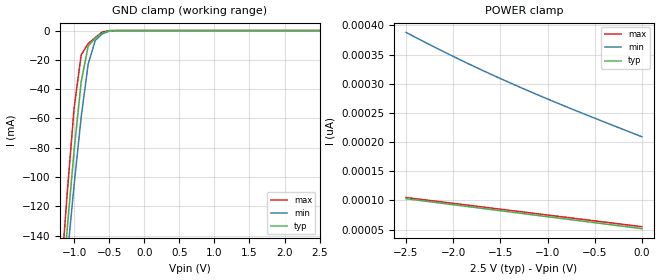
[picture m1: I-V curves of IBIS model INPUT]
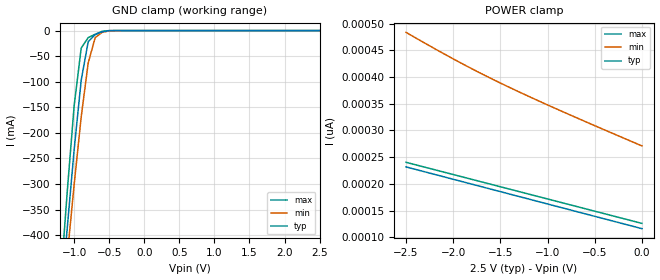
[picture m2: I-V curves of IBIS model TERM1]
|   PERICOM SEMICONDUCTOR CORP
|   IBIS Model of PI3C32X245
|   Product Family: 3C
|   BQSOP (B) Package
[IBIS Ver] 3.2
[Comment char] |_char
[File Name] pi3c32x245_b_25v.ibs
[File Rev] 2.0
[Source] File originated at Pericom Semiconductor Corp.
[Date] 03/15/18
[Disclaimer] (C) Copyright PERICOM Semiconductor Corporation
   All rights reserved
  Pericom Semiconductor Corporation hereby grants the user of
  this IBIS model a non-exclusive, nontransferable license to
  use this IBIS model under the following terms.
  This IBIS model is provided on an "AS IS" basis and Pericom
  makes absolutely no warranty with respect to the information
  contained herein. PERICOM DISCLAIMS AND CUSTOMER WAIVES ALL
  WARRANTIES, EXPRESSED OR IMPLIED, INCLUDING WARRANTIES OF
  MERCHANTABILITY OR FITNESS FOR A PARTICULAR PURPOSE. The
  entire risk as to quality and performance is with the customer.
  Accordingly, in no event shall the company be liable for any
  damages, whether in contract or tort, including any lost
  profits or other incidental, consequential, exemplary, or
  punitive damages arising out of the use or application of the
  IBIS model provided in this package. Further, Pericom reserves
  the right to make changes without notice to any product herein
  to improve reliability, function, or design. Pericom does not
  convey any license under patent rights or any other intellectual
  property rights, including those of third parties.
  The user is granted this license only to use the IBIS model
  and is not granted rights to sell, load, rent, lease or license
  the IBIS model in whole or in part, or in modified form to anyone
  other than user. User may modify the IBIS model to suit its specific
  application but rights to derivative works and such modifications
  shall belong to Pericom.
  Pericom is not obligated to provide maintenance or support
  for the licensed IBIS model.
  Contact Pericom at ATTN: APPLICATION ENGINEERING / IBIS MODELS
  2380 Bering Drive, San Jose, CA 95131
[Component] PI3C32X245
[Manufacturer] Pericom Semiconductor Corp.
[Package]
| Variable   typ   min   max
R_pkg   0.03818ohm   0.02666ohm   0.04970ohm
L_pkg   0.79246nH   0.73792nH   0.84700nH
C_pkg   0.19953pF   0.16164pF   0.23742pF
[Pin]  signal_name   model_name   R_pin   L_pin   C_pin
1   NC   NC   0.04970   0.84700nH   0.23742pF
2   A0   TERM1   0.04714   0.83488nH   0.22900pF
3   A1   TERM1   0.04458   0.82276nH   0.22058pF
4   A2   TERM1   0.04202   0.81064nH   0.21216pF
5   A3   TERM1   0.03946   0.79852nH   0.20374pF
6   A4   TERM1   0.03690   0.78640nH   0.19532pF
7   A5   TERM1   0.03434   0.77428nH   0.18690pF
8   A6   TERM1   0.03178   0.76216nH   0.17848pF
9   A7   TERM1   0.02922   0.75004nH   0.17006pF
10   GND   GND   0.02666   0.73792nH   0.16164pF
11   NC   NC   0.02666   0.73792nH   0.16164pF
12   A8   TERM1   0.02922   0.75004nH   0.17006pF
13   A9   TERM1   0.03178   0.76216nH   0.17848pF
14   A10   TERM1   0.03434   0.77428nH   0.18690pF
15   A11   TERM1   0.03690   0.78640nH   0.19532pF
16   A12   TERM1   0.03946   0.79852nH   0.20374pF
17   A13   TERM1   0.04202   0.81064nH   0.21216pF
18   A14   TERM1   0.04458   0.82276nH   0.22058pF
19   A15   TERM1   0.04714   0.83488nH   0.22900pF
20   GND   GND   0.04970   0.84700nH   0.23742pF
21   B15   TERM2   0.04970   0.84700nH   0.23742pF
22   B14   TERM2   0.04714   0.83488nH   0.22900pF
23   B13   TERM2   0.04458   0.82276nH   0.22058pF
24   B12   TERM2   0.04202   0.81064nH   0.21216pF
25   B11   TERM2   0.03946   0.79852nH   0.20374pF
26   B10   TERM2   0.03690   0.78640nH   0.19532pF
27   B9   TERM2   0.03434   0.77428nH   0.18690pF
28   B8   TERM2   0.03178   0.76216nH   0.17848pF
29   _BE2   INPUT   0.02922   0.75004nH   0.17006pF
30   VCC   POWER   0.02666   0.73792nH   0.16164pF
31   B7   TERM2   0.02666   0.73792nH   0.16164pF
32   B6   TERM2   0.02922   0.75004nH   0.17006pF
33   B5   TERM2   0.03178   0.76216nH   0.17848pF
34   B4   TERM2   0.03434   0.77428nH   0.18690pF
35   B3   TERM2   0.03690   0.78640nH   0.19532pF
36   B2   TERM2   0.03946   0.79852nH   0.20374pF
37   B1   TERM2   0.04202   0.81064nH   0.21216pF
38   B0   TERM2   0.04458   0.82276nH   0.22058pF
39   _BE1   INPUT   0.04714   0.83488nH   0.22900pF
40   VCC   POWER   0.04970   0.84700nH   0.23742pF
[Series Switch Groups]
On 1 /
Off 2 /
[Series Pin Mapping]   pin_2   model_name  function_table_group
2   38   SWITCH1   1
3   37   SWITCH1   1
4   36   SWITCH1   1
5   35   SWITCH1   1
6   34   SWITCH1   1
7   33   SWITCH1   1
8   32   SWITCH1   1
9   31   SWITCH1   1
12   28   SWITCH1   2
13   27   SWITCH1   2
14   26   SWITCH1   2
15   25   SWITCH1   2
16   24   SWITCH1   2
17   23   SWITCH1   2
18   22   SWITCH1   2
19   21   SWITCH1   2
|   Model SWITCH1
[Model] SWITCH1
Model_type Series_switch
| variable   typ   min   max
C_comp   10.000pF   9.800pF   10.200pF
[Voltage Range]   2.5000V   2.2500V   2.7500V
[GND Clamp Reference]   0.0000V   0.0000V   0.0000V
[POWER Clamp Reference]   2.5000V   2.2500V   2.7500V
[Temperature Range]   25   85   -40
[On]
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[OFF]
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| Models and submodels in the file (4): INPUT (Input), SWITCH1 (Series_switch), TERM1 (Terminator), TERM2 (Terminator)
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|   Model INPUT
[Model] INPUT
Model_type Input
Vinl = 750mV
Vinh = 1.80V
| variable   typ   min   max
C_comp   3.500pF   3.400pF   3.600pF
[Voltage Range]   2.5000V   2.2500V   2.7500V
[GND Clamp Reference]   0.0000V   0.0000V   0.0000V
[POWER Clamp Reference]   2.5000V   2.2500V   2.7500V
[Temperature Range]   25   85   -40
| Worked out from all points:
|   GND clamp passes 1 mA (typ) near -0.56 V on its own axis
[GND Clamp]
| Voltage   I(typ)   I(min)   I(max)
-2.5V     -998.2mA   -927.2mA   -1.099A
-1.2V     -193.5mA   -207.1mA   -176.6mA
-1.1V     -135.8mA   -155mA     -111.4mA
-1V       -81.33mA   -105mA     -52.61mA
-900mV    -34.92mA   -59.01mA   -16.58mA
-800mV    -10.56mA   -22.8mA    -8.882mA
-700mV    -5.104mA   -6.74mA    -4.717mA
-600mV    -1.611mA   -2.212mA   -981.9uA
-500mV    -145.9uA   -381.4uA   -24.42uA
-400mV    -4.329uA   -29.72uA   -133.6nA
2.5V      51.65pA    224.9pA    50pA
[POWER Clamp]   |Note: Vtable = Vcc - Voutput
| Voltage   I(typ)   I(min)   I(max)
-2.5V     103.1pA    388pA      105pA
-2V       92.73pA    346.8pA    95pA
-1.7V     86.54pA    323.7pA    89pA
-1.4V     80.36pA    301.7pA    83pA
-800mV    68.04pA    260.5pA    71pA
0V        51.65pA    209.1pA    55pA
|   Model TERM1
[Model] TERM1
Model_type Terminator
| variable   typ   min   max
C_comp   5.000pF   4.900pF   5.100pF
[Voltage Range]   2.5000V   2.2500V   2.7500V
[GND Clamp Reference]   0.0000V   0.0000V   0.0000V
[POWER Clamp Reference]   2.5000V   2.2500V   2.7500V
[Temperature Range]   25   85   -40
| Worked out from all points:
|   GND clamp passes 1 mA (typ) near -0.54 V on its own axis
[GND Clamp]
| Voltage   I(typ)   I(min)   I(max)
-2.5V     -2.832A    -2.628A    -3.121A
-1.2V     -551.9mA   -590.4mA   -503.2mA
-1.1V     -387.8mA   -442.8mA   -316.8mA
-1V       -232.2mA   -300.6mA   -146.4mA
-900mV    -97.23mA   -169.1mA   -34.28mA
-800mV    -21.65mA   -63.17mA   -13.78mA
-700mV    -7.82mA    -13.64mA   -7.205mA
-600mV    -2.298mA   -3.355mA   -1.407mA
-500mV    -202.1uA   -564.7uA   -32.57uA
2.5V      116pA      289.9pA    114.4pA
[POWER Clamp]   |Note: Vtable = Vcc - Voutput
| Voltage   I(typ)   I(min)   I(max)
-2.5V     231.7pA    483.7pA    240.3pA
-2V       208.5pA    434.1pA    217.4pA
-1.5V     185.4pA    388.8pA    194.5pA
-900mV    157.6pA    339.9pA    167.1pA
0V        116pA      271pA      125.9pA
